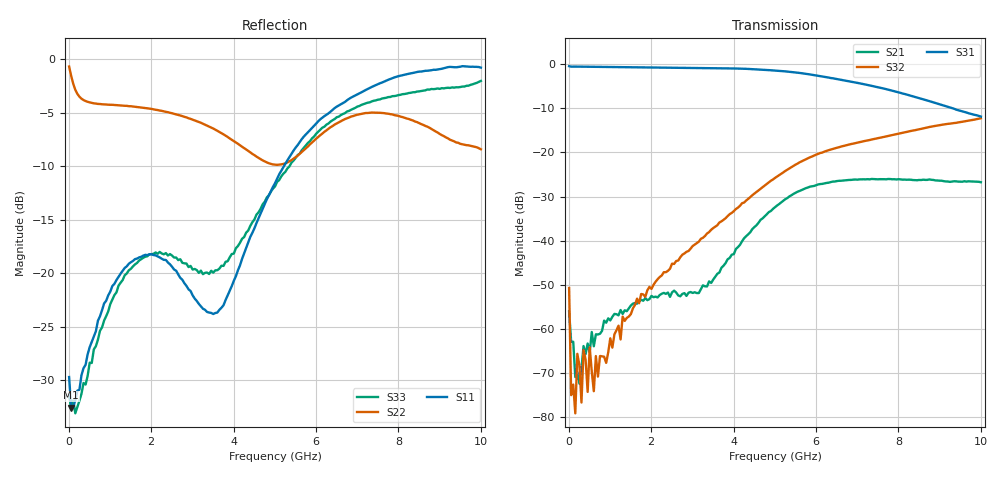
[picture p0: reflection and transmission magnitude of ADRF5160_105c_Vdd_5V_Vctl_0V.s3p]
! Device:  ADRF5160
! Description: Silicon SPDT Switch
! Frequency:  0.7 -  4 GHz
! Ports:
!	RFc	= Port 1
!	RF1	= Port 2
!  RF2  = Port 3
! Vdd:  5 Volt
! Control:  0 Volt
! Data:  Data was collected using a calibrated 4 port network analyzer and de-embedded using Agilent's AFR De-Embedding.
! Note:  Analog Devices supplies this data as a sample of measured data
!  for this product.  Your particular data for this product may vary.
!  Data was taken at 105 degrees C.
!S3P File: Measurements: <S11,S12,S13>,
!<S21,S22,S23>,
!<S31,S32,S33>:
# Hz S  dB  R 50
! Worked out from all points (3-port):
!   201 points, 10 MHz to 10 GHz, reference 50 ohm
!   strongest paths, dB at 10 MHz, 2.507 GHz, 5.005 GHz, 7.503 GHz, 10 GHz:
!     S31: -0.5, -0.8, -1.4, -5.2, -11.9
!     S32: -50.7, -45.2, -25.8, -16.8, -12.3
!     S21: -56.0, -51.7, -32.4, -26.1, -26.7
!   lowest |S11| = -32.5 dB at 59.95 MHz (marker M1), VSWR 1.05, Z = 52.4 - j0.502 ohm
!   |S11| at or under -10 dB: start of sweep to 5.219 GHz
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1e7  -29.68 11.3  -58.34 -13.4  -0.51 -0.3
     -56.02 -68.0  -0.68 -8.4  -51.73 -77.8
     -0.47 -0.1  -50.70 -13.2  -31.31 -8.9
5.995e7  -32.54 -11.7  -65.24 -98.9  -0.56 -1.8
         -62.89 174.4  -1.55 -45.3  -79.39 55.8
         -0.57 -1.6  -74.96 25.4  -32.71 -9.3
1.5985e8  -31.84 -33.7  -87.47 -32.4  -0.56 -4.3
          -70.87 25.9  -2.85 -94.1  -70.74 5.8
          -0.56 -4.4  -79.08 3.8  -33.07 -33.8
2.098e8  -30.95 -39.5  -63.69 72.0  -0.57 -5.6
         -69.73 72.7  -3.23 -109.9  -65.73 42.3
         -0.57 -5.7  -65.60 -91.0  -32.49 -41.1
2.5975e8  -30.86 -49.3  -77.96 147.5  -0.59 -6.9
          -72.37 79.2  -3.50 -121.7  -62.13 6.4
          -0.57 -6.8  -68.22 93.2  -31.90 -45.1
5.5945e8  -26.40 -71.2  -64.21 87.3  -0.60 -14.8
          -60.66 87.7  -4.07 -158.2  -77.34 -46.0
          -0.60 -14.8  -69.62 -80.7  -28.37 -80.7
6.5935e8  -25.40 -79.1  -60.40 84.9  -0.60 -17.5
          -61.19 88.5  -4.14 -164.7  -67.95 -65.8
          -0.61 -17.4  -66.11 -131.8  -26.80 -89.4
5.005e9  -11.58 22.2  -32.43 99.4  -1.44 -137.4
         -32.41 99.5  -9.84 103.2  -25.77 111.8
         -1.45 -137.3  -25.77 111.4  -11.88 -130.0
7.4026e9  -2.49 -41.8  -26.01 -11.8  -5.03 150.0
          -26.02 -11.8  -4.98 76.7  -16.98 12.6
          -5.03 150.0  -16.98 12.7  -3.88 158.8
1e10  -0.78 -75.8  -26.77 -86.4  -11.89 91.8
      -26.75 -86.4  -8.41 0.7  -12.25 -75.3
      -11.88 91.8  -12.26 -75.2  -2.02 79.8
